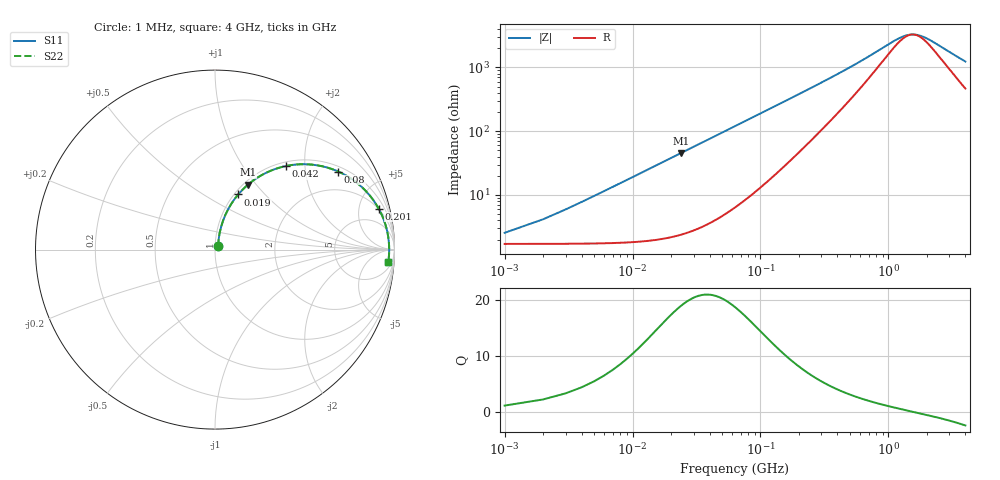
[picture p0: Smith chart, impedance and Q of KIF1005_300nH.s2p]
!version-2
!date-12.2020
!Series
# MHz S RI R 50
!Freq ReS11 ImS11 ReS21 ImS21 ReS12 ImS12 ReS22 ImS22
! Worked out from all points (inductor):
!   4000 points, 1 MHz to 4 GHz, reference 50 ohm
!   read as one part in series: L = 302 nH near 21 MHz
!   highest Q = 18.7 at 24 MHz (marker M1), where L = 302 nH
!   self-resonance near 1.55 GHz
!   S11 on the Smith chart (normalised r, x): 1 MHz: 1.03, +0.04; 19 MHz: 1.04, +0.72; 42 MHz: 1.08, +1.59; 80 MHz: 1.18, +3.03; 201 MHz: 1.94, +7.62; 4 GHz: 10, -23
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1  0.0171 0.0183  0.9829 -0.0183  0.9829 -0.0183  0.0171 0.0183
19  0.1293 0.3073  0.8707 -0.3073  0.8707 -0.3073  0.1293 0.3073
24  0.1845 0.3626  0.8155 -0.3626  0.8155 -0.3626  0.1845 0.3626
32  0.279 0.4251  0.721 -0.4251  0.721 -0.4251  0.279 0.4251
42  0.3935 0.4653  0.6065 -0.4653  0.6065 -0.4653  0.3935 0.4653
61  0.5689 0.4697  0.4311 -0.4697  0.4311 -0.4697  0.5689 0.4697
80  0.6869 0.4348  0.3131 -0.4348  0.3131 -0.4348  0.6869 0.4348
101  0.7706 0.3871  0.2294 -0.3871  0.2294 -0.3871  0.7706 0.3871
127  0.8338 0.3331  0.1662 -0.3331  0.1662 -0.3331  0.8338 0.3331
159  0.8791 0.2799  0.1209 -0.2799  0.1209 -0.2799  0.8791 0.2799
201  0.9118 0.2285  0.0882 -0.2285  0.0882 -0.2285  0.9118 0.2285
285  0.9413 0.1636  0.0587 -0.1636  0.0587 -0.1636  0.9413 0.1636
389  0.9555 0.1181  0.0445 -0.1181  0.0445 -0.1181  0.9555 0.1181
516  0.9628 0.0851  0.0372 -0.0851  0.0372 -0.0851  0.9628 0.0851
668  0.9666 0.0605  0.0334 -0.0605  0.0334 -0.0605  0.9666 0.0605
1020  0.9697 0.0277  0.0303 -0.0277  0.0303 -0.0277  0.9697 0.0277
1334  0.9704 0.0097  0.0296 -0.0097  0.0296 -0.0097  0.9704 0.0097
1620  0.9705 -0.00282  0.0295 0.00282  0.0295 0.00282  0.9705 -0.00282
2001  0.9702 -0.0166  0.0298 0.0166  0.0298 0.0166  0.9702 -0.0166
2667  0.9691 -0.0365  0.0309 0.0365  0.0309 0.0365  0.9691 -0.0365
3334  0.9675 -0.054  0.0325 0.054  0.0325 0.054  0.9675 -0.054
4000  0.9654 -0.0701  0.0346 0.0701  0.0346 0.0701  0.9654 -0.0701
